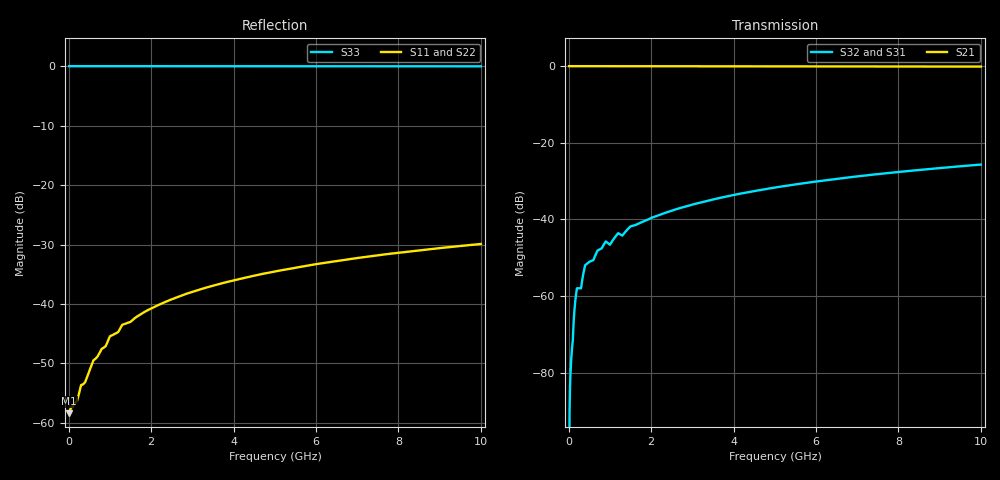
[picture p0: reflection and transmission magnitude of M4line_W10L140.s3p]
! Created Fri Sep 09 13:58:18 2011
# ghz S ma R 50
! 3 Port Network Data from SP1.SP block
! freq  magS11  angS11  magS12  angS12  magS13  angS13
!  magS21  angS21
!  magS22  angS22  magS23  angS23
!  magS31  angS31  magS32  angS32
!  magS33  angS33
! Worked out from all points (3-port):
!   1000 points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, 10 MHz to 10 GHz, reference 50 ohm
!   strongest paths, dB at 10 MHz, 2.51 GHz, 5.01 GHz, 7.51 GHz, 10 GHz:
!     S21: 0.0, 0.0, -0.1, -0.1, -0.1
!     S32: -, -37.7, -31.7, -28.2, -25.7
!     S31: -, -37.7, -31.7, -28.2, -25.7
!   lowest |S11| = -58.4 dB at 10 MHz (marker M1), VSWR 1.00, Z = 50.1 + j0.00779 ohm
!   |S11| at or under -10 dB: start of sweep to end of sweep
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0.01  0.001205 3.7  0.9988 -0.0  0 0.0
      0.9988 -0.0  0.001205 3.7  0 0.0
      0 0.0  0 0.0  1 0.0
0.06  0.001344 15.7  0.9987 -0.0  0.0001481 90.0
      0.9987 -0.0  0.001344 15.7  0.0001481 90.0
      0.0001481 90.0  0.0001481 90.0  1 -0.0
0.16  0.001475 29.8  0.9987 -0.1  0.0008667 89.9
      0.9987 -0.1  0.001475 29.8  0.0008667 89.9
      0.0008667 89.9  0.0008667 89.9  1 -0.1
0.21  0.001568 37.4  0.9988 -0.1  0.001267 89.9
      0.9988 -0.1  0.001568 37.4  0.001267 89.9
      0.001267 89.9  0.001267 89.9  1 -0.1
0.43  0.002347 54.7  0.9986 -0.3  0.002613 89.8
      0.9986 -0.3  0.002347 54.7  0.002613 89.8
      0.002613 89.8  0.002613 89.8  1 -0.3
0.88  0.004378 66.3  0.9982 -0.5  0.004979 89.6
      0.9982 -0.5  0.004378 66.3  0.004979 89.6
      0.004979 89.6  0.004979 89.6  1 -0.6
1.32  0.006728 69.8  0.9977 -0.7  0.00636 89.5
      0.9977 -0.7  0.006728 69.8  0.00636 89.5
      0.00636 89.5  0.00636 89.5  1 -0.7
2.35  0.01043 69.1  0.9963 -1.3  0.01224 88.8
      0.9963 -1.3  0.01043 69.1  0.01224 88.8
      0.01224 88.8  0.01224 88.8  0.9998 -1.4
5.01  0.01882 68.1  0.9929 -2.5  0.02608 87.7
      0.9929 -2.5  0.01882 68.1  0.02608 87.7
      0.02608 87.7  0.02608 87.7  0.9993 -3.0
10  0.03199 66.4  0.9864 -4.7  0.05197 85.4
    0.9864 -4.7  0.03199 66.4  0.05197 85.4
    0.05197 85.4  0.05197 85.4  0.9971 -6.0
